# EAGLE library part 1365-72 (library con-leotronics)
DUAL ROW STRAIGHT HEADER 1364 SERIES. 1.27mm x 1.27mm. Without Fixing Post. SMT Source: http://www.leotronics.co.uk/Conexcon/Data%20Sheets/sec.%20A/1364ing.pdf
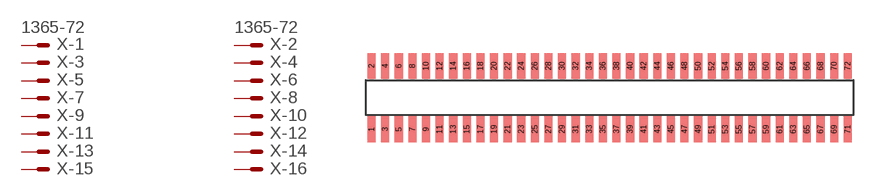
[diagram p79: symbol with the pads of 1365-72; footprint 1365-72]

Designator prefix X; gates -1=MVAL -2=MVAL -3=M -4=M -5=M -6=M -7=M -8=M -9=M -10=M -11=M -12=M -13=M -14=M -15=M -16=M -17=M -18=M -19=M -20=M -21=M -22=M -23=M -24=M -25=M -26=M -27=M -28=M -29=M -30=M -31=M -32=M -33=M -34=M -35=M -36=M -37=M -38=M -39=M -40=M -41=M -42=M -43=M -44=M -45=M -46=M -47=M -48=M -49=M -50=M -51=M -52=M -53=M -54=M -55=M -56=M -57=M -58=M -59=M -60=M -61=M -62=M -63=M -64=M -65=M -66=M -67=M -68=M -69=M -70=M -71=M -72=M

## 1365-72 (OC_FARNELL: unknown; OC_NEWARK: unknown)  [1365-72]
1  -1:S  pas
2  -2:S  pas
3  -3:S  pas
4  -4:S  pas
5  -5:S  pas
6  -6:S  pas
7  -7:S  pas
8  -8:S  pas
9  -9:S  pas
10  -10:S  pas
11  -11:S  pas
12  -12:S  pas
13  -13:S  pas
14  -14:S  pas
15  -15:S  pas
16  -16:S  pas
17  -17:S  pas
18  -18:S  pas
19  -19:S  pas
20  -20:S  pas
21  -21:S  pas
22  -22:S  pas
23  -23:S  pas
24  -24:S  pas
25  -25:S  pas
26  -26:S  pas
27  -27:S  pas
28  -28:S  pas
29  -29:S  pas
30  -30:S  pas
31  -31:S  pas
32  -32:S  pas
33  -33:S  pas
34  -34:S  pas
35  -35:S  pas
36  -36:S  pas
37  -37:S  pas
38  -38:S  pas
39  -39:S  pas
40  -40:S  pas
41  -41:S  pas
42  -42:S  pas
43  -43:S  pas
44  -44:S  pas
45  -45:S  pas
46  -46:S  pas
47  -47:S  pas
48  -48:S  pas
49  -49:S  pas
50  -50:S  pas
51  -51:S  pas
52  -52:S  pas
53  -53:S  pas
54  -54:S  pas
55  -55:S  pas
56  -56:S  pas
57  -57:S  pas
58  -58:S  pas
59  -59:S  pas
60  -60:S  pas
61  -61:S  pas
62  -62:S  pas
63  -63:S  pas
64  -64:S  pas
65  -65:S  pas
66  -66:S  pas
67  -67:S  pas
68  -68:S  pas
69  -69:S  pas
70  -70:S  pas
71  -71:S  pas
72  -72:S  pas

## Footprint 1365-72 (pad centres in mm)
DUAL ROW STRAIGHT HEADER 1364 SERIES. 1.27mm x 1.27mm. Without Fixing Post. SMT Source: http://www.leotronics.co.uk/Conexcon/Data%20Sheets/sec.%20A/1364ing.pdf
smd 0.76 x 2.4: 1 -22.225,-2.95; 2 -22.225,2.95; 3 -20.955,-2.95; 4 -20.955,2.95; 5 -19.685,-2.95; 6 -19.685,2.95; 7 -18.415,-2.95; 8 -18.415,2.95; 9 -17.145,-2.95; 10 -17.145,2.95; 11 -15.875,-2.95; 12 -15.875,2.95; 13 -14.605,-2.95; 14 -14.605,2.95; 15 -13.335,-2.95; 16 -13.335,2.95; 17 -12.065,-2.95; 18 -12.065,2.95; 19 -10.795,-2.95; 20 -10.795,2.95; 21 -9.525,-2.95; 22 -9.525,2.95; 23 -8.255,-2.95; 24 -8.255,2.95; 25 -6.985,-2.95; 26 -6.985,2.95; 27 -5.715,-2.95; 28 -5.715,2.95; 29 -4.445,-2.95; 30 -4.445,2.95; 31 -3.175,-2.95; 32 -3.175,2.95; 33 -1.905,-2.95; 34 -1.905,2.95; 35 -0.635,-2.95; 36 -0.635,2.95; 37 0.635,-2.95; 38 0.635,2.95; 39 1.905,-2.95; 40 1.905,2.95; 41 3.175,-2.95; 42 3.175,2.95; 43 4.445,-2.95; 44 4.445,2.95; 45 5.715,-2.95; 46 5.715,2.95; 47 6.985,-2.95; 48 6.985,2.95; 49 8.255,-2.95; 50 8.255,2.95; 51 9.525,-2.95; 52 9.525,2.95; 53 10.795,-2.95; 54 10.795,2.95; 55 12.065,-2.95; 56 12.065,2.95; 57 13.335,-2.95; 58 13.335,2.95; 59 14.605,-2.95; 60 14.605,2.95; 61 15.875,-2.95; 62 15.875,2.95; 63 17.145,-2.95; 64 17.145,2.95; 65 18.415,-2.95; 66 18.415,2.95; 67 19.685,-2.95; 68 19.685,2.95; 69 20.955,-2.95; 70 20.955,2.95; 71 22.225,-2.95; 72 22.225,2.95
